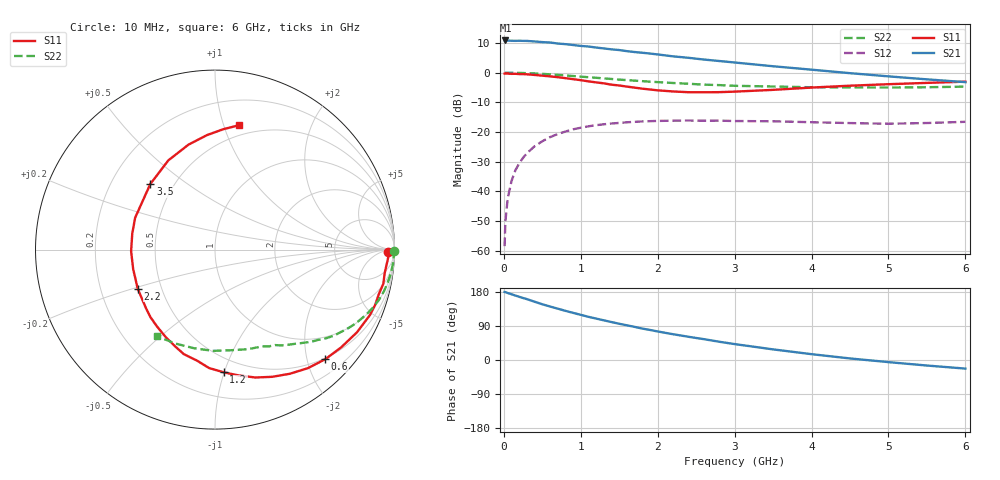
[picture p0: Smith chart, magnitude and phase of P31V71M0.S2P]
! SIEMENS Small Signal Semiconductors
! BFP181
! Si NPN RF Bipolar Junction Transistor in SOT143
! VCE = 1.75 V  IC = 1 mA
! Common Emitter S-Parameters:  March  1996
# GHz  S  MA  R  50
!  f  S11  S21  S12  S22
! GHz  MAG  ANG  MAG  ANG  MAG  ANG  MAG  ANG
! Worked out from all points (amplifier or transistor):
!   36 points, 10 MHz to 6 GHz, reference 50 ohm
!   highest |S21| = 10.8 dB at 20 MHz (marker M1)
!   |S21| within 3 dB of that: start of sweep to 1.401 GHz
!   unconditionally stable (mu >= 1): 2.986 GHz to end of sweep
!   at 250 MHz: K = 0.10, MSG = 19.7 dB, |S12| = -28.7 dB
!   at 1.4 GHz: K = 0.51, MSG = 12.5 dB, |S12| = -17.1 dB
!   at 6 GHz: K = 1.29, MAG = 3.5 dB, |S12| = -16.6 dB
!   S11 on the Smith chart (normalised r, x): 10 MHz: 46, -19; 600 MHz: 0.48, -2.34; 1.2 GHz: 0.39, -1.00; 2.2 GHz: 0.37, -0.21; 3.5 GHz: 0.37, +0.37; 6 GHz: 0.41, +1.13
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0.01  0.9634 -0.9  3.471 179.6  0.0012 79.9  0.999 -0.3
0.02  0.9686 -1.5  3.482 179.2  0.0031 91.7  0.991 -0.7
0.05  0.9636 -3.5  3.462 176.8  0.0076 90.2  0.9964 -1.8
0.1  0.9545 -7.8  3.438 173.5  0.015 84.3  0.9962 -3.6
0.15  0.9569 -11.5  3.429 170.1  0.0227 81.6  0.9928 -5.3
0.3  0.937 -22.9  3.418 160.7  0.044 74.9  0.9803 -10.6
0.4  0.9155 -30.2  3.35 153.7  0.0577 70.4  0.9694 -13.9
0.6  0.866 -44.9  3.217 141.2  0.082 60.6  0.9362 -20.4
0.8  0.8079 -58.9  3.017 129.8  0.102 52.4  0.8968 -26.0
1.1  0.7131 -79.4  2.753 113.9  0.1249 41.3  0.8374 -33.3
1.2  0.6856 -85.9  2.645 109.3  0.1305 37.8  0.8198 -35.7
1.5  0.6078 -106.6  2.401 95.6  0.1425 29.5  0.7626 -41.3
1.8  0.5372 -126.8  2.161 82.9  0.1509 22.9  0.7191 -46.1
2.2  0.4825 -153.2  1.88 68.0  0.1554 15.1  0.6696 -52.3
2.4  0.4686 -166.7  1.778 61.3  0.1564 11.8  0.6502 -55.2
2.8  0.4695 169.1  1.57 48.2  0.1556 6.7  0.6173 -60.9
3  0.479 158.3  1.482 42.0  0.1533 4.5  0.6005 -63.9
3.5  0.5133 134.6  1.281 28.0  0.1518 0.6  0.5844 -71.7
4  0.561 117.6  1.122 15.4  0.1464 -1.9  0.5678 -81.0
4.5  0.603 104.2  0.98 4.1  0.1416 -3.7  0.5643 -91.3
5.5  0.6722 86.1  0.771 -14.6  0.142 -0.4  0.568 -112.8
6  0.7055 79.1  0.692 -22.7  0.1487 0.2  0.5816 -124.0
